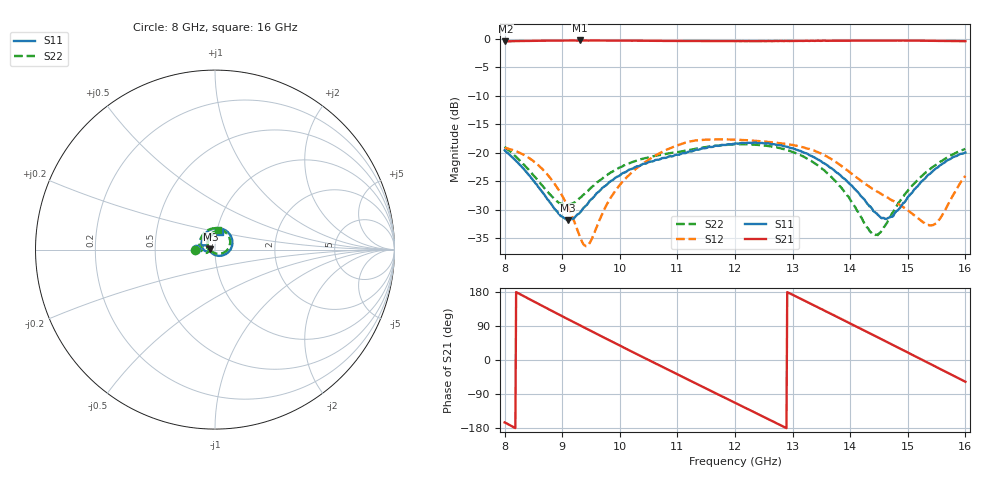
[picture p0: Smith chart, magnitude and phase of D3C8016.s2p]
! 11/6/2020 8:36:23 AM
! C:\USERS\KOBYR\DESKTOP\8.0 - 16.0 GHZ (D3I8016).S2P
! CHANNEL.1
! TR.MEASUREMENT
! CORRECTED.DATA
# GHZ S RI R 50.0
! FREQ.GHZ  S11RE  S11IM  S21RE  S21IM  S12RE  S12IM  S22RE  S22IM
!; PortSelection: Port_12
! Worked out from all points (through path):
!   601 points, 8 GHz to 16 GHz, reference 50 ohm
!   highest |S21| = -0.29 dB at 9.307 GHz (marker M1); lowest = -0.5 dB at 8.013 GHz (marker M2)
!   lowest |S11| = -31.8 dB at 9.093 GHz (marker M3), VSWR 1.05, Z = 47.5 + j0.225 ohm
!   |S11| at or under -10 dB: start of sweep to end of sweep
!   |S22| runs from -34.4 to -18.5 dB; largest |S21 - S12| = 0.98
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8  -0.1054 0.00496  -0.9162 -0.2489  -0.0252 0.1079  -0.1131 -0.00451
8.013333  -0.1036 0.00599  -0.9193 -0.2358  -0.0227 0.108  -0.1115 -0.00432
8.52  -0.0503 0.0233  -0.8595 0.4285  0.0511 0.0653  -0.0601 0.0159
9.093333  -0.0257 0.00237  -0.3015 0.9187  0.0338 0.00465  -0.0347 -0.00423
9.306667  -0.0291 -0.00648  -0.0251 0.9674  0.0178 0.00476  -0.038 -0.0132
9.346667  -0.0307 -0.00785  0.0268 0.9648  0.0153 0.00613  -0.0392 -0.0146
9.48  -0.0367 -0.0107  0.1986 0.9466  0.0101 0.0128  -0.0449 -0.0177
10.06667  -0.0667 0.00318  0.8092 0.5252  0.0387 0.0422  -0.0774 -0.00386
10.66667  -0.0738 0.0464  0.9371 -0.2088  0.0977 -0.00732  -0.0858 0.0409
11.37333  -0.0468 0.0958  0.391 -0.8715  0.0359 -0.1242  -0.0616 0.0908
11.68  -0.023 0.1128  0.0188 -0.9536  -0.0308 -0.1277  -0.0391 0.1089
12  0.0105 0.1203  -0.3693 -0.8787  -0.0894 -0.0953  -0.00749 0.1185
12.70667  0.0816 0.0854  -0.9277 -0.233  -0.1174 0.0363  0.0649 0.0911
13.01333  0.0964 0.0512  -0.9463 0.1476  -0.0815 0.0836  0.0825 0.0588
13.34667  0.0923 0.0116  -0.7965 0.5391  -0.0225 0.1033  0.0809 0.02
14.01333  0.0404 -0.0331  -0.0899 0.9596  0.0481 0.0457  0.0302 -0.0227
14.4  0.00253 -0.0308  0.3951 0.8805  0.0448 0.0177  -0.00515 -0.0186
14.66667  -0.0209 -0.017  0.6773 0.6881  0.0395 0.00665  -0.0255 -0.00422
15  -0.0386 0.0134  0.9083 0.3281  0.0312 -0.0015  -0.04 0.0236
15.32  -0.0377 0.0483  0.9589 -0.0813  0.0236 -0.000544  -0.0393 0.0553
15.53333  -0.0261 0.0709  0.8945 -0.3496  0.0248 0.00592  -0.0295 0.0763
16  0.0306 0.0959  0.5143 -0.8038  0.0628 -0.00399  0.0194 0.1064
